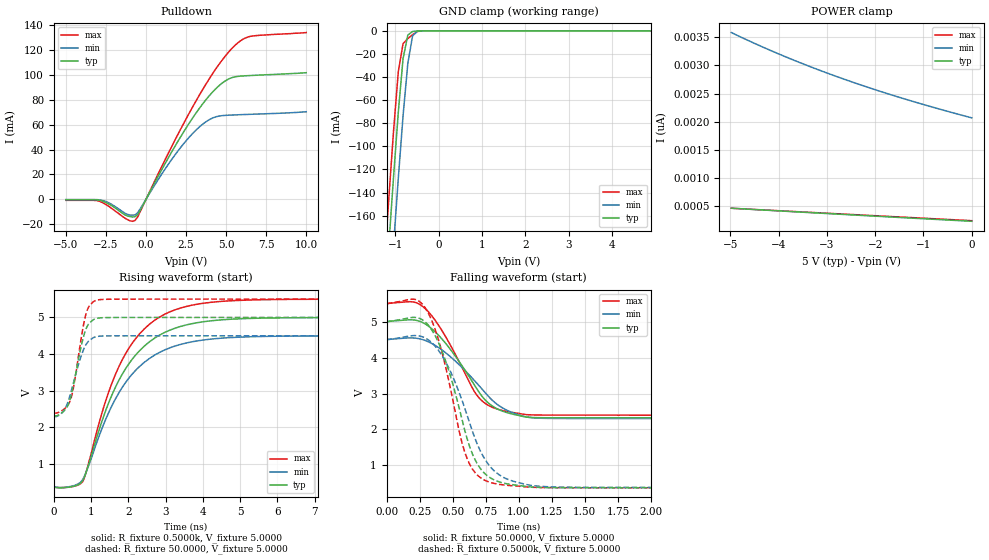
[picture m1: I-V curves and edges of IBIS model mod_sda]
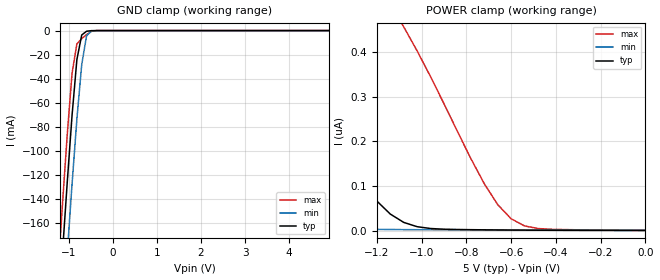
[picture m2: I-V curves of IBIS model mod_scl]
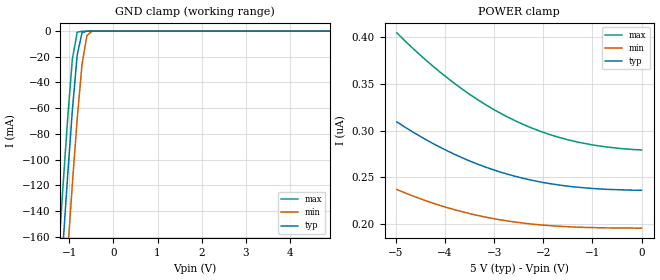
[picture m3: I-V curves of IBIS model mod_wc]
| IBIS (I/O, Buffer, Information, Specification) Model, officially
| electronic behavioral standard for Buffer structures of digital pins.
[IBIS ver]  4.0
[File name] m24c16_g3_tssop8.ibs
[File Rev]  1.0
[Date]   24 March 2015
[Source]   CAD & Design Services (Catania) - STMicroelectronics
[Notes]
   (Note1)  This IBIS model includes the TSSOP8 package data
   (Note2)  This IBIS model has some Notes about the non-monotonicity
   of the I-V curves, but they are not indicative of problems
   inside the model;
[Copyright] (c) 2015 STMicroelectronics
|   Component M24C16
[Component] M24C16
[Manufacturer] STMicroelectronics
[Package]
| variable   typ   min   max
R_pkg   0.0   0.0   0.0
L_pkg   0.0H   0.0H   0.0H
C_pkg   0.0F   0.0F   0.0F
[Pin]  signal_name   model_name   R_pin   L_pin   C_pin
1   NC   NC   NA   NA   NA
2   NC   NC   NA   NA   NA
3   NC   NC   NA   NA   NA
4   VSS   GND   NA   NA   NA
5   SDA   mod_sda   NA   NA   NA
6   SCL   mod_scl   NA   NA   NA
7   WCN   mod_wc   NA   NA   NA
8   VCC   POWER   NA   NA   NA
[Package Model]  182696_TSSOP8
[Define Package Model]  182696_TSSOP8
[Manufacturer]  STMicroelectronics
[OEM]  STMicroelectronics
[Description]  8 pin TSSOP package
[Number Of Pins]  8
[Pin Numbers]
|Pin Num   Terminal Name
1   | net1
2   | net2
3   | net3
4   | net4_GND
5   | net5
6   | net6
7   | net7
8   | net8_VDD
[Model Data]
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[End Model Data]
[End Package Model]
| Models and submodels in the file (3): mod_sda (I/O_open_drain), mod_scl (Input), mod_wc (Input)
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|   Model mod_sda
[Model]   mod_sda
Model_type I/O_open_drain
Polarity   Non-Inverting
Vinl   =   1.500V
Vinh   =   3.500V
Vmeas  =   2.500V
Cref   =   10pF
Rref   =   1k
Vref   =   5.000V
C_comp   2.668pF   2.547pF   2.925pF
[Temperature Range]  25.0000   0.1050k   -40.0000
[Voltage Range]   5.0000V   4.5000V   5.5000V
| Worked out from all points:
|   slope of the pulldown table from 0 to 0.75 V, typ, clamps not added: 41 ohm
|   GND clamp passes 1 mA (typ) near -0.62 V on its own axis
|   rising waveform, R_fixture 0.5000k, V_fixture 5.0000: 20-80 % time 1.26ns typ, 1.29ns min, 1.21ns max; typ from 0.375 V to 5 V
|   rising waveform, R_fixture 50.0000, V_fixture 5.0000: 20-80 % time 333ps typ, 379ps min, 299ps max; typ from 2.32 V to 5 V
|   falling waveform, R_fixture 50.0000, V_fixture 5.0000: 20-80 % time 306ps typ, 350ps min, 274ps max; typ from 5 V to 2.32 V
|   falling waveform, R_fixture 0.5000k, V_fixture 5.0000: 20-80 % time 221ps typ, 263ps min, 195ps max; typ from 5 V to 0.375 V
[Pulldown]
|Voltage   I(typ)   I(min)   I(max)
-5V       -312.2uA   -165uA     -763.5uA
-2.92V    -677.1uA   -343.3uA   -1.424mA
-1.16V    -13.26mA   -12.03mA   -16.18mA
-680mV    -13.89mA   -12.4mA    -16.87mA
-360mV    -8.955mA   -7.564mA   -9.806mA
1.56V     37.05mA    31.19mA    41.24mA
2.84V     63.92mA    51.88mA    72.48mA
4.12V     85.6mA     65.04mA    100.1mA
5.24V     97.05mA    67.58mA    119.4mA
5.88V     98.83mA    67.92mA    127mA
6.52V     99.35mA    68.23mA    130.8mA
10V       101.6mA    70.29mA    133.8mA
[GND_clamp]
|Voltage   I(typ)   I(min)   I(max)
-5V       -2.463A    -2.517A    -2.427A
-1.26V    -247.9mA   -307.9mA   -207.4mA
-1.15V    -186.5mA   -246.4mA   -146mA
-1.04V    -126.9mA   -186.2mA   -87.22mA
-930mV    -70.75mA   -128mA     -35.65mA
-820mV    -24.14mA   -73.68mA   -11.1mA
-710mV    -3.674mA   -28.28mA   -6.723mA
-600mV    -555.3uA   -4.336mA   -3.311mA
-490mV    -79.08uA   -420.4uA   -612.8uA
-380mV    -6.392uA   -66.66uA   -6.41uA
4.9V      226.1pA    2.161nA    215.1pA
[POWER_clamp]
|Voltage   I(typ)   I(min)   I(max)
-4.98V    463.1pA    3.584nA    462.4pA
-4.44V    437pA      3.369nA    438.2pA
-3.84V    408.3pA    3.148nA    411.5pA
-3.3V     382.8pA    2.963nA    387.5pA
-2.7V     354.6pA    2.773nA    360.9pA
-2.1V     326.7pA    2.597nA    334.3pA
-1.44V    296.3pA    2.418nA    305.1pA
-720mV    263.3pA    2.237nA    273.3pA
0V        230.6pA    2.069nA    241.5pA
[Ramp]
| variable   typ   min   max
dV/dt_r   1.6064/0.3695n   1.2928/0.4314n   1.8610/0.3311n
dV/dt_f   1.6064/0.3364n   1.2928/0.3810n   1.8610/0.2932n
R_load = 50.0000
[Rising Waveform]
R_fixture= 0.5000k
V_fixture= 5.0000   | New Temp 105 (min)
V_fixture_min= 4.5000
V_fixture_max= 5.5000
|time   V(typ)   V(min)   V(max)
0s        375.3mV    388.2mV    378mV
510ps     387.6mV    402.4mV    387.5mV
770ps     535.3mV    567.6mV    514.5mV
1.39ns    2.45V      2.212V     2.715V
1.79ns    3.366V     3.015V     3.748V
2.29ns    4.08V      3.652V     4.537V
2.99ns    4.598V     4.12V      5.094V
3.69ns    4.826V     4.332V     5.331V
4.67ns    4.947V     4.446V     5.45V
10ns      5V         4.5V       5.5V
[Rising Waveform]
R_fixture= 50.0000
V_fixture= 5.0000   | new Temp 105 (min)
V_fixture_min= 4.5000
V_fixture_max= 5.5000
|time   V(typ)   V(min)   V(max)
0s        2.323V     2.304V     2.398V
270ps     2.445V     2.465V     2.495V
370ps     2.584V     2.669V     2.6V
450ps     2.81V      2.928V     2.756V
530ps     3.169V     3.228V     3.098V
730ps     4.191V     3.936V     4.4V
850ps     4.648V     4.234V     5.042V
950ps     4.841V     4.368V     5.308V
1.13ns    4.969V     4.473V     5.464V
10ns      5V         4.5V       5.5V
[Falling Waveform]
R_fixture= 50.0000
V_fixture= 5.0000   | New Temp 105 (min)
V_fixture_min= 4.5000
V_fixture_max= 5.5000
|time   V(typ)   V(min)   V(max)
0s        5V         4.5V       5.5V
200ps     5.049V     4.546V     5.548V
280ps     4.961V     4.491V     5.402V
360ps     4.742V     4.355V     5.075V
460ps     4.335V     4.095V     4.496V
640ps     3.379V     3.459V     3.213V
700ps     3.033V     3.215V     2.876V
840ps     2.567V     2.689V     2.564V
1.06ns    2.345V     2.345V     2.412V
10ns      2.323V     2.304V     2.398V
[Falling Waveform]
R_fixture= 0.5000k
V_fixture= 5.0000   | New Temp 105 (min)
V_fixture_min= 4.5000
V_fixture_max= 5.5000
|time   V(typ)   V(min)   V(max)
0s        5V         4.5V       5.5V
200ps     5.119V     4.61V      5.626V
290ps     4.998V     4.549V     5.398V
430ps     4.079V     3.989V     3.991V
550ps     2.584V     3.019V     1.938V
610ps     1.733V     2.388V     1.181V
710ps     909.7mV    1.397V     658.9mV
870ps     522.3mV    696.2mV    463mV
1.37ns    377.7mV    394mV      379.5mV
10ns      375.3mV    388.2mV    378mV
|   Model mod_scl
[Model]   mod_scl
Model_type Input
Vinl   =   1.500V
Vinh   =   3.500V
C_comp   2.119pF   2.024pF   2.323pF
[Temperature Range]  25.0000   0.1050k   -40.0000
[Voltage Range]   5.0000V   4.5000V   5.5000V
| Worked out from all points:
|   GND clamp passes 1 mA (typ) near -0.62 V on its own axis
[GND_clamp]
|Voltage   I(typ)   I(min)   I(max)
-5V       -2.463A    -2.517A    -2.427A
-1.26V    -247.9mA   -307.9mA   -207.4mA
-1.15V    -186.5mA   -246.4mA   -146mA
-1.04V    -126.9mA   -186.2mA   -87.22mA
-930mV    -70.75mA   -128mA     -35.65mA
-820mV    -24.14mA   -73.68mA   -11.1mA
-710mV    -3.674mA   -28.28mA   -6.723mA
-600mV    -555.3uA   -4.336mA   -3.311mA
-490mV    -79.08uA   -420.4uA   -612.8uA
-380mV    -6.392uA   -66.66uA   -6.41uA
4.9V      226.1pA    2.161nA    215.1pA
[POWER_clamp]
|Voltage   I(typ)   I(min)   I(max)
-4.98V    41.7uA     36.31uA    47.97uA
-2.52V    6.697uA    450.4nA    21.91uA
-2.22V    1.719uA    344.2nA    12.84uA
-1.74V    451.4nA    84.33nA    2.356uA
-1.62V    376nA      35.7nA     840.7nA
-1.5V     288.5nA    11.54nA    683.2nA
-1.26V    104.1nA    3.055nA    588.5nA
-1.08V    18.31nA    2.156nA    456.3nA
-720mV    1.675nA    1.244nA    104.9nA
-600mV    1.178nA    1.077nA    26.35nA
-480mV    836.1pA    950.9pA    4.582nA
0V        246.5pA    681.8pA    582.1pA
|   Model mod_wc
[Model]   mod_wc
Model_type Input
Vinl   =   1.500V
Vinh   =   3.500V
C_comp   2.119pF   2.024pF   2.323pF
[Temperature Range]  25.0000   0.1050k   -40.0000
[Voltage Range]   5.0000V   4.5000V   5.5000V
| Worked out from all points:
|   GND clamp passes 1 mA (typ) near -0.70 V on its own axis
[GND_clamp]
|Voltage   I(typ)   I(min)   I(max)
-5V       -2.311A    -2.366A    -2.271A
-1.26V    -228mA     -288.4mA   -182.4mA
-1.15V    -170.3mA   -230.5mA   -124.7mA
-1.04V    -114.2mA   -173.9mA   -69.64mA
-930mV    -61.71mA   -119.1mA   -21.79mA
-820mV    -18.53mA   -68.08mA   -895uA
-710mV    -1.148mA   -25.53mA   -96.19uA
-600mV    -54.23uA   -3.496mA   -58.44uA
-490mV    -13.42uA   -208.3uA   -29.04uA
4.9V      235.9nA    191.1nA    278.2nA
[POWER_clamp]
|Voltage   I(typ)   I(min)   I(max)
-4.98V    309.2nA    236.8nA    404.6nA
-4.38V    290nA      224.6nA    375nA
-3.78V    273.9nA    214.8nA    349.4nA
-3.48V    267nA      210.8nA    338.1nA
-3.18V    260.9nA    207.3nA    327.9nA
-2.58V    251.1nA    202nA      310.7nA
-2.04V    244.7nA    198.8nA    298.8nA
-1.74V    242.1nA    197.7nA    293.6nA
-1.38V    239.7nA    196.7nA    288.6nA
-840mV    237.4nA    195.8nA    283.3nA
-420mV    236.5nA    195.5nA    280.7nA
0V        236nA      195.4nA    279.2nA
